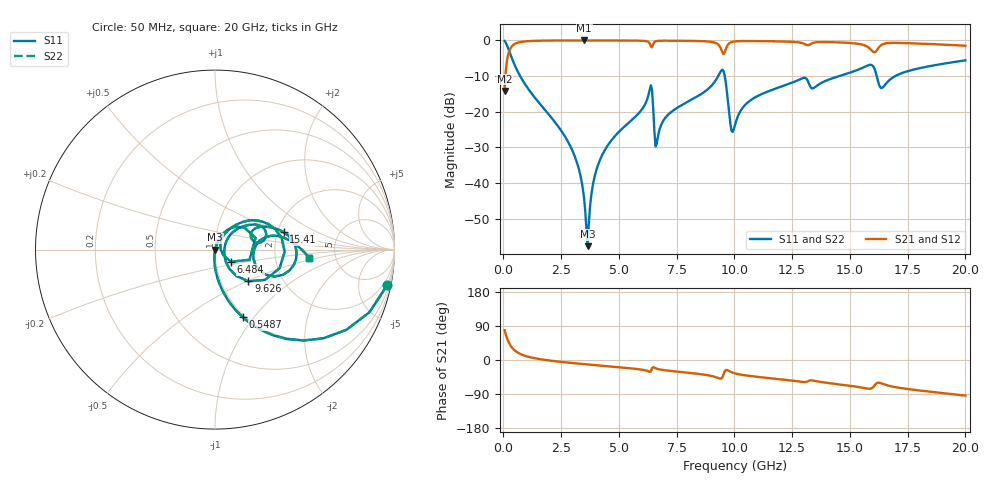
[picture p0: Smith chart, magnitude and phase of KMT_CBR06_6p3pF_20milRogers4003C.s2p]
! Data measured by Modelithics Inc. support@modelithics.com 813-866-6335
! KEMET CBR0603 6.3pF, Pad Width= 0.851mm, Pad Length= 0.64mm, Pad Gap= 0.62mm, 20mil Rogers 4003C substrate Data, January 2022
# hz S ma R 50
! 2 Port Network Data from SP1.SP block
! freq  magS11  angS11  magS21  angS21  magS12  angS12  magS22  angS22
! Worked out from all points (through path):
!   401 points, 50 MHz to 20 GHz, reference 50 ohm
!   highest |S21| = -0.01 dB at 3.491 GHz (marker M1); lowest = -14.2 dB at 50 MHz (marker M2)
!   group delay of S21, straight-line fit = 14.5 ps
!   lowest |S11| = -57.7 dB at 3.641 GHz (marker M3), VSWR 1.00, Z = 50.1 - j0.00928 ohm
!   |S11| at or under -10 dB: 722.9 MHz to 9.298 GHz (8.575 GHz wide, 171 % of centre); 9.582 GHz to 14.54 GHz (4.954 GHz wide, 41.1 % of centre); 16.16 GHz to 16.96 GHz (801.7 MHz wide, 4.84 % of centre)
!   |S22| runs from -57.7 to -0.2 dB; largest |S21 - S12| = 0
!   S11 on the Smith chart (normalised r, x): 50 MHz: 0.97, -9.87; 548.8 MHz: 0.97, -0.88; 6.484 GHz: 1.18, -0.16; 9.626 GHz: 1.35, -0.51; 15.41 GHz: 2.17, +0.49; 20 GHz: 3.16, -0.40
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5e7  0.9806 -11.5  0.1959 78.5  0.1959 78.5  0.9806 -11.5
2.495e8  0.7065 -45.8  0.7072 44.1  0.7072 44.1  0.7065 -45.8
5.4875e8  0.4074 -67.6  0.9126 22.3  0.9126 22.3  0.4074 -67.6
2.74325e9  0.04072 -95.0  0.998 -6.5  0.998 -6.5  0.04072 -95.0
3.391625e9  0.01025 -93.4  0.9986 -10.4  0.9986 -10.4  0.01025 -93.4
3.491375e9  0.006099 -89.0  0.9986 -10.9  0.9986 -10.9  0.006099 -89.0
3.641e9  0.001305 -4.1  0.9986 -11.8  0.9986 -11.8  0.001305 -4.1
3.94025e9  0.01206 70.1  0.9984 -13.4  0.9984 -13.4  0.01206 70.1
4.389125e9  0.02902 71.3  0.9979 -15.8  0.9979 -15.8  0.02902 71.3
6.33425e9  0.2047 37.0  0.9059 -31.3  0.9059 -31.3  0.2047 37.0
6.483875e9  0.1112 -37.4  0.8938 -18.8  0.8938 -18.8  0.1112 -37.4
6.73325e9  0.05251 53.2  0.9873 -24.6  0.9873 -24.6  0.05251 53.2
9.177125e9  0.2718 36.9  0.9243 -44.9  0.9243 -44.9  0.2718 36.9
9.626e9  0.2565 -43.5  0.7516 -26.4  0.7516 -26.4  0.2565 -43.5
9.875375e9  0.05396 -18.3  0.9472 -32.3  0.9472 -32.3  0.05396 -18.3
1.0025e10  0.06537 28.0  0.9686 -35.3  0.9686 -35.3  0.06537 28.0
1.107238e10  0.1704 42.7  0.9782 -45.1  0.9782 -45.1  0.1704 42.7
1.336662e10  0.212 17.4  0.9113 -53.9  0.9113 -53.9  0.212 17.4
1.54115e10  0.3956 14.1  0.8898 -71.8  0.8898 -71.8  0.3956 14.1
1.610975e10  0.3634 -24.4  0.6925 -64.1  0.6925 -64.1  0.3634 -24.4
1.670825e10  0.2771 13.2  0.9206 -68.4  0.9206 -68.4  0.2771 13.2
2e10  0.5255 -5.0  0.8413 -94.0  0.8413 -94.0  0.5255 -5.0
